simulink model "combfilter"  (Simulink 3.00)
settings: Solver=FixedStepDiscrete  SolverMode=SingleTasking  StartTime=0.0  StopTime=4  RelTol=1e-3

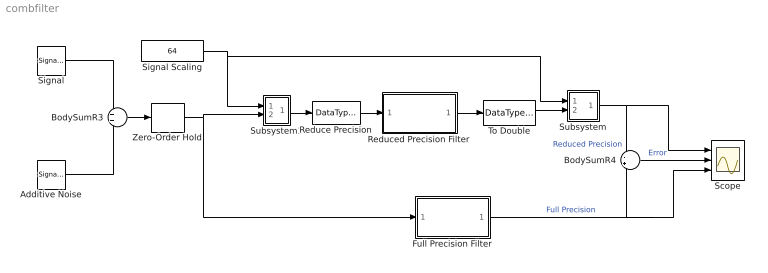
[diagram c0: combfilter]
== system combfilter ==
  Additive Noise : SignalGenerator  WaveForm=sine  Amplitude=3  Frequency=25  Units=Hertz
  BodySumR3 : Sum  Inputs=++  SaturateOnIntegerOverflow=on
  BodySumR4 : Sum  Inputs=-+  SaturateOnIntegerOverflow=on
  Full Precision Filter : Subsystem
  Reduce Precision : DataTypeConversion  DataType=single  SaturateOnIntegerOverflow=on
  Reduced Precision Filter : Subsystem
  Scope : Scope  NumInputPorts=3
  Signal : SignalGenerator  WaveForm=sine  Amplitude=100  Frequency=1  Units=Hertz
  Signal Scaling : Constant  Value=64
  Subsystem : Subsystem
  Subsystem1 : Subsystem
  To Double : DataTypeConversion  DataType=double  SaturateOnIntegerOverflow=on
  Zero-Order Hold : ZeroOrderHold  SampleTime=0.01
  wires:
  Reduced Precision Filter/1(Output) -> To Double/1
  Subsystem1/1(Out1) -> Reduce Precision/1
  To Double/1 -> Subsystem/2(In2)
  Zero-Order Hold/1 -> Subsystem1/2(In2), Full Precision Filter/1(Input)
  Subsystem/1(Out1) -> Scope/1, BodySumR4/1  "Reduced Precision"
  Reduce Precision/1 -> Reduced Precision Filter/1(Input)
  Signal Scaling/1 -> Subsystem/1(In1), Subsystem1/1(In1)
  Signal/1 -> BodySumR3/1
  Additive Noise/1 -> BodySumR3/2
  BodySumR3/1 -> Zero-Order Hold/1
  BodySumR4/1 -> Scope/2  "Error"
  Full Precision Filter/1(Output) -> Scope/3, BodySumR4/2  "Full Precision"

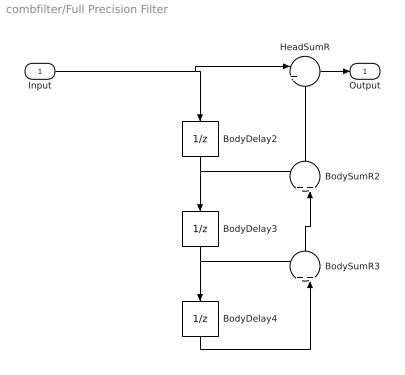
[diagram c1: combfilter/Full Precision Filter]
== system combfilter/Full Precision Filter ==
  Input : Inport  Port=1  PortWidth=-1  SampleTime=-1  DataType=auto
  BodyDelay2 : UnitDelay  Orientation=down  X0=0  SampleTime=-1
  BodyDelay3 : UnitDelay  Orientation=down  X0=0  SampleTime=-1
  BodyDelay4 : UnitDelay  Orientation=down  X0=0  SampleTime=-1
  BodySumR2 : Sum  Orientation=up  Inputs=++|  SaturateOnIntegerOverflow=on
  BodySumR3 : Sum  Orientation=up  Inputs=++|  SaturateOnIntegerOverflow=on
  HeadSumR : Sum  Inputs=|++  SaturateOnIntegerOverflow=on
  Output : Outport  Port=1
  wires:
  Input/1 -> BodyDelay2/1, HeadSumR/1
  BodyDelay2/1 -> BodyDelay3/1, BodySumR2/1
  BodyDelay3/1 -> BodyDelay4/1, BodySumR3/1
  BodyDelay4/1 -> BodySumR3/2
  BodySumR2/1 -> HeadSumR/2
  BodySumR3/1 -> BodySumR2/2
  HeadSumR/1 -> Output/1

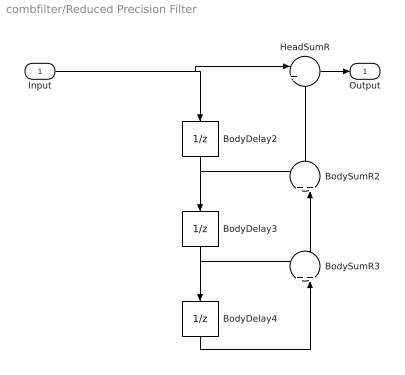
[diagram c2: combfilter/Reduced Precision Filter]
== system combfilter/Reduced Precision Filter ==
  Input : Inport  Port=1  PortWidth=-1  SampleTime=-1  DataType=auto
  BodyDelay2 : UnitDelay  Orientation=down  X0=0  SampleTime=-1
  BodyDelay3 : UnitDelay  Orientation=down  X0=0  SampleTime=-1
  BodyDelay4 : UnitDelay  Orientation=down  X0=0  SampleTime=-1
  BodySumR2 : Sum  Orientation=up  Inputs=++|  SaturateOnIntegerOverflow=on
  BodySumR3 : Sum  Orientation=up  Inputs=++|  SaturateOnIntegerOverflow=on
  HeadSumR : Sum  Inputs=|++  SaturateOnIntegerOverflow=on
  Output : Outport  Port=1
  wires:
  HeadSumR/1 -> Output/1
  BodySumR3/1 -> BodySumR2/2
  BodySumR2/1 -> HeadSumR/2
  BodyDelay4/1 -> BodySumR3/2
  BodyDelay3/1 -> BodySumR3/1, BodyDelay4/1
  BodyDelay2/1 -> BodySumR2/1, BodyDelay3/1
  Input/1 -> HeadSumR/1, BodyDelay2/1

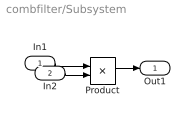
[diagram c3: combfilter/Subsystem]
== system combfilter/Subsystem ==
  In1 : Inport  Port=1  PortWidth=-1  SampleTime=-1  DataType=auto
  In2 : Inport  Port=2  PortWidth=-1  SampleTime=-1  DataType=auto
  Product : Product  Inputs=/*  SaturateOnIntegerOverflow=on
  Out1 : Outport  Port=1
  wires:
  In1/1 -> Product/1
  Product/1 -> Out1/1
  In2/1 -> Product/2

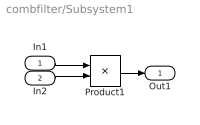
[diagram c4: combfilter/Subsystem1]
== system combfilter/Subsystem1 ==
  In1 : Inport  Port=1  PortWidth=-1  SampleTime=-1  DataType=auto
  In2 : Inport  Port=2  PortWidth=-1  SampleTime=-1  DataType=auto
  Product1 : Product  Inputs=2  SaturateOnIntegerOverflow=on
  Out1 : Outport  Port=1
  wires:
  In2/1 -> Product1/2
  In1/1 -> Product1/1
  Product1/1 -> Out1/1
